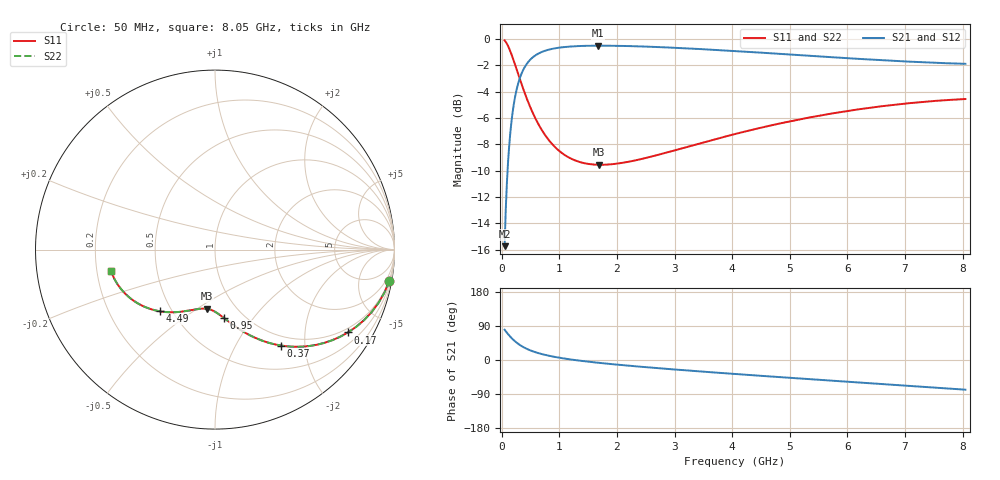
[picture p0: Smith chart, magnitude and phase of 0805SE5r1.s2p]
! AVX Thin Film Operation		Date: August 2001
! Description: Accu-P® Series, Thin Film, SMD, RF Capacitor
! Part Number: 08051J5R1ABT
! 50 MHz  -  8.05 GHz
! Serial Measurements
# mhz S db R 50
!	S11		S21		S12		S22
!	dB	Phase	dB	Phase	dB	Phase	dB	Phase
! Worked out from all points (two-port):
!   401 points, 50 MHz to 8.05 GHz, reference 50 ohm
!   highest |S21| = -0.51 dB at 1.67 GHz (marker M1); lowest = -15.7 dB at 50 MHz (marker M2)
!   |S21| within 3 dB of the highest: 277.7 MHz to end of sweep
!   lowest |S11| = -9.6 dB at 1.69 GHz (marker M3), VSWR 2.00, Z = 37.1 - j27.6 ohm
!   |S11| at or under -10 dB: nowhere
!   |S22| runs from -9.6 to -0.1 dB; largest |S21 - S12| = 9.3e-05
!   S11 on the Smith chart (normalised r, x): 50 MHz: 1, -11; 170 MHz: 0.85, -3.30; 370 MHz: 0.84, -1.56; 950 MHz: 0.81, -0.73; 4.49 GHz: 0.43, -0.38; 8.05 GHz: 0.26, -0.10
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50  -0.12 -10.2  -15.73 79.8  -15.73 79.8  -0.12 -10.2
90  -0.37 -18.0  -10.90 72.0  -10.90 72.0  -0.37 -18.0
110  -0.54 -21.7  -9.34 68.3  -9.34 68.3  -0.54 -21.7
130  -0.73 -25.3  -8.09 64.7  -8.09 64.7  -0.73 -25.3
170  -1.18 -31.9  -6.24 58.1  -6.24 58.1  -1.18 -31.9
250  -2.20 -43.1  -4.01 46.9  -4.01 46.9  -2.20 -43.1
310  -2.99 -49.8  -3.03 40.2  -3.03 40.2  -2.99 -49.8
370  -3.75 -55.5  -2.38 34.5  -2.38 34.5  -3.75 -55.5
490  -5.12 -64.2  -1.60 25.8  -1.60 25.8  -5.12 -64.2
610  -6.25 -70.6  -1.18 19.3  -1.18 19.3  -6.25 -70.6
770  -7.41 -77.1  -0.87 12.9  -0.87 12.9  -7.41 -77.1
950  -8.32 -82.6  -0.69 7.3  -0.69 7.3  -8.32 -82.6
1390  -9.39 -92.3  -0.54 -2.4  -0.54 -2.4  -9.39 -92.3
1670  -9.55 -97.1  -0.51 -7.2  -0.51 -7.2  -9.55 -97.1
1690  -9.56 -97.4  -0.51 -7.5  -0.51 -7.5  -9.56 -97.5
2170  -9.35 -104.5  -0.54 -14.5  -0.54 -14.5  -9.35 -104.5
2730  -8.78 -111.7  -0.62 -21.8  -0.62 -21.8  -8.78 -111.7
4050  -7.22 -126.8  -0.92 -36.9  -0.92 -36.9  -7.22 -126.8
4490  -6.75 -131.5  -1.04 -41.6  -1.04 -41.6  -6.75 -131.5
5390  -5.93 -140.9  -1.29 -51.0  -1.29 -51.0  -5.93 -140.9
6730  -5.04 -154.6  -1.65 -64.7  -1.65 -64.7  -5.04 -154.6
8050  -4.57 -168.2  -1.89 -78.3  -1.89 -78.3  -4.57 -168.2
